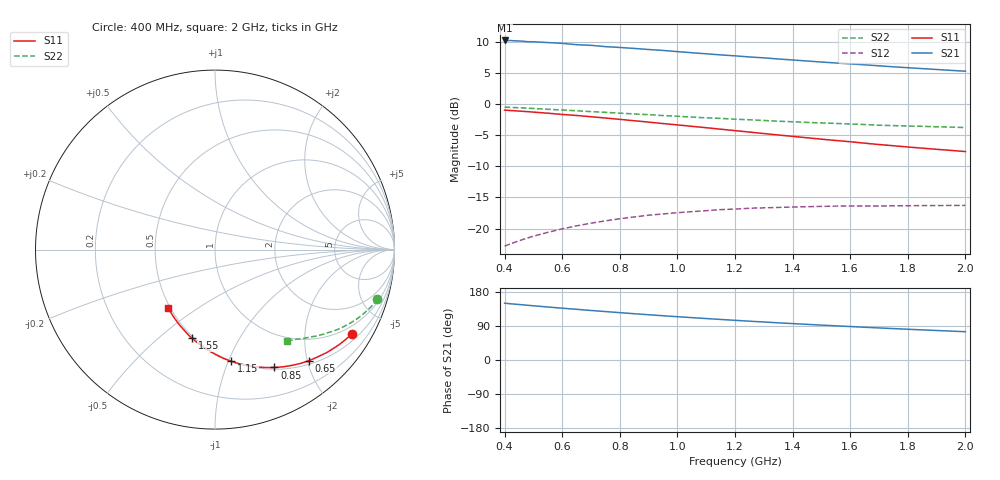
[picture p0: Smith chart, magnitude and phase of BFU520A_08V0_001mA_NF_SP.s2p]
! Filename:  P:\Prog\Test\Noise\ATS_data\Testdata_Net\06 Compressed Noise after Statistics\BFU520A_APG2013_30_A05_08p0V_001mA_NF_CM01_D.sf
! Date/Time: Wed 24/Apr/2013 20:06:19
! BFU520A_APG2013_30_A05_08p0V_1to20mA_NF_CM01_Bias1_R.sf
! Noise Parameter Data File
! BFU520A_APG2013_30_A05_08p0V_1to20mA_NF_CM01
! Date/time: Thu Apr 11 09:33:54 2013
! freq range =  0.4000 to  2.0000 GHz, 37 points
! bias range =  1.0000 to 19.9950 mA, 8 points
! bias supplies used: 1 1 0 0 0 0
! VAR bias_mode= 1  ! Specify V_out, I_out
! VAR bias_var = 1  ! Bias variable = I_out
! VAR V_out= 8.000000
! VAR I_out= 1.000000
! VAR V_in= 0.791600
! VAR I_in= 0.010400
! Device data file deembeded for feedlines and parallel
! Original file: \06 Compressed Noise after Statistics\BFU520A_APG2013_30_A05_08p0V_001mA_NF_CM01_R.sf
! Feed-files: PR017V01_150413_Feed1.s2p, PR017V01_150413_Feed2.s2p
! Parallel-file: PR017V01_150413_Par.s2p
# MHz S MA R 50
!  Freq-MHz  S11-mag  S11-arg  S21-mag  S21-arg  S12-mag  S12-arg  S22-mag  S22-arg
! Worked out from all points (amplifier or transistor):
!   37 points, 400 MHz to 2 GHz, reference 50 ohm
!   highest |S21| = 10.2 dB at 400 MHz (marker M1)
!   |S21| within 3 dB of that: start of sweep to 1.358 GHz
!   unconditionally stable (mu >= 1): nowhere
!   at 500 MHz: K = 0.23, MSG = 15.6 dB, |S12| = -21.2 dB
!   at 1.1 GHz: K = 0.48, MSG = 12.6 dB, |S12| = -17.1 dB
!   at 2 GHz: K = 0.86, MSG = 10.8 dB, |S12| = -16.3 dB
!   lowest NFmin = 0.51 dB at 440 MHz
!   S11 on the Smith chart (normalised r, x): 400 MHz: 0.72, -3.39; 650 MHz: 0.56, -2.03; 850 MHz: 0.52, -1.50; 1.15 GHz: 0.50, -1.03; 1.55 GHz: 0.49, -0.65; 2 GHz: 0.49, -0.38
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400  0.895 -31.6  3.249 149.9  0.07226 69.7  0.9462 -16.9
420  0.8892 -33.2  3.245 148.4  0.07537 68.8  0.9417 -17.7
440  0.883 -34.7  3.225 147.1  0.07831 67.9  0.9374 -18.4
460  0.8764 -36.2  3.209 145.8  0.0813 67.1  0.9333 -19.1
480  0.8705 -37.6  3.175 144.4  0.08409 66.2  0.9275 -19.9
500  0.863 -39.1  3.17 143.1  0.08686 65.4  0.9229 -20.6
550  0.846 -42.8  3.125 139.8  0.09333 63.3  0.9094 -22.3
600  0.8265 -46.4  3.079 136.7  0.09946 61.4  0.8969 -23.9
650  0.8112 -49.7  3.003 133.8  0.1053 59.6  0.8847 -25.5
700  0.792 -53.3  2.968 130.7  0.1105 57.9  0.8713 -27.0
750  0.774 -56.5  2.898 127.8  0.1154 56.3  0.8591 -28.4
850  0.7354 -63.2  2.803 122.1  0.1241 53.2  0.8343 -31.1
950  0.6981 -69.6  2.701 116.8  0.1311 50.6  0.8097 -33.6
1050  0.6635 -75.7  2.588 111.8  0.1369 48.4  0.7867 -35.8
1150  0.6292 -81.7  2.487 107.0  0.1421 46.3  0.7682 -37.8
1200  0.6127 -84.7  2.444 104.7  0.1436 45.5  0.7568 -38.8
1350  0.5653 -93.2  2.307 98.1  0.1479 43.4  0.7293 -41.6
1500  0.523 -101.7  2.18 92.1  0.1508 41.8  0.7064 -44.1
1550  0.5106 -104.4  2.142 90.2  0.1516 41.5  0.7001 -45.0
1750  0.4633 -115.5  1.995 82.9  0.1525 41.1  0.6723 -48.0
1850  0.443 -120.8  1.93 79.5  0.1531 41.2  0.6633 -49.5
2000  0.416 -128.9  1.839 74.7  0.1536 42.2  0.649 -51.7
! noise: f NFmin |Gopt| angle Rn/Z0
400  0.6072  0.6006  17.37  0.3638
460  0.6134  0.628  21.15  0.3794
600  0.6437  0.6103  24.04  0.3656
800  0.6379  0.5856  38.42  0.2867
1000  0.6511  0.5994  49.23  0.2667
1200  0.72  0.6118  58.37  0.2691
1400  0.7544  0.5847  68.56  0.2232
1600  0.7046  0.5645  81.64  0.1845
1800  0.6883  0.4939  96.52  0.1377
2000  0.7368  0.4693  106.4  0.134
